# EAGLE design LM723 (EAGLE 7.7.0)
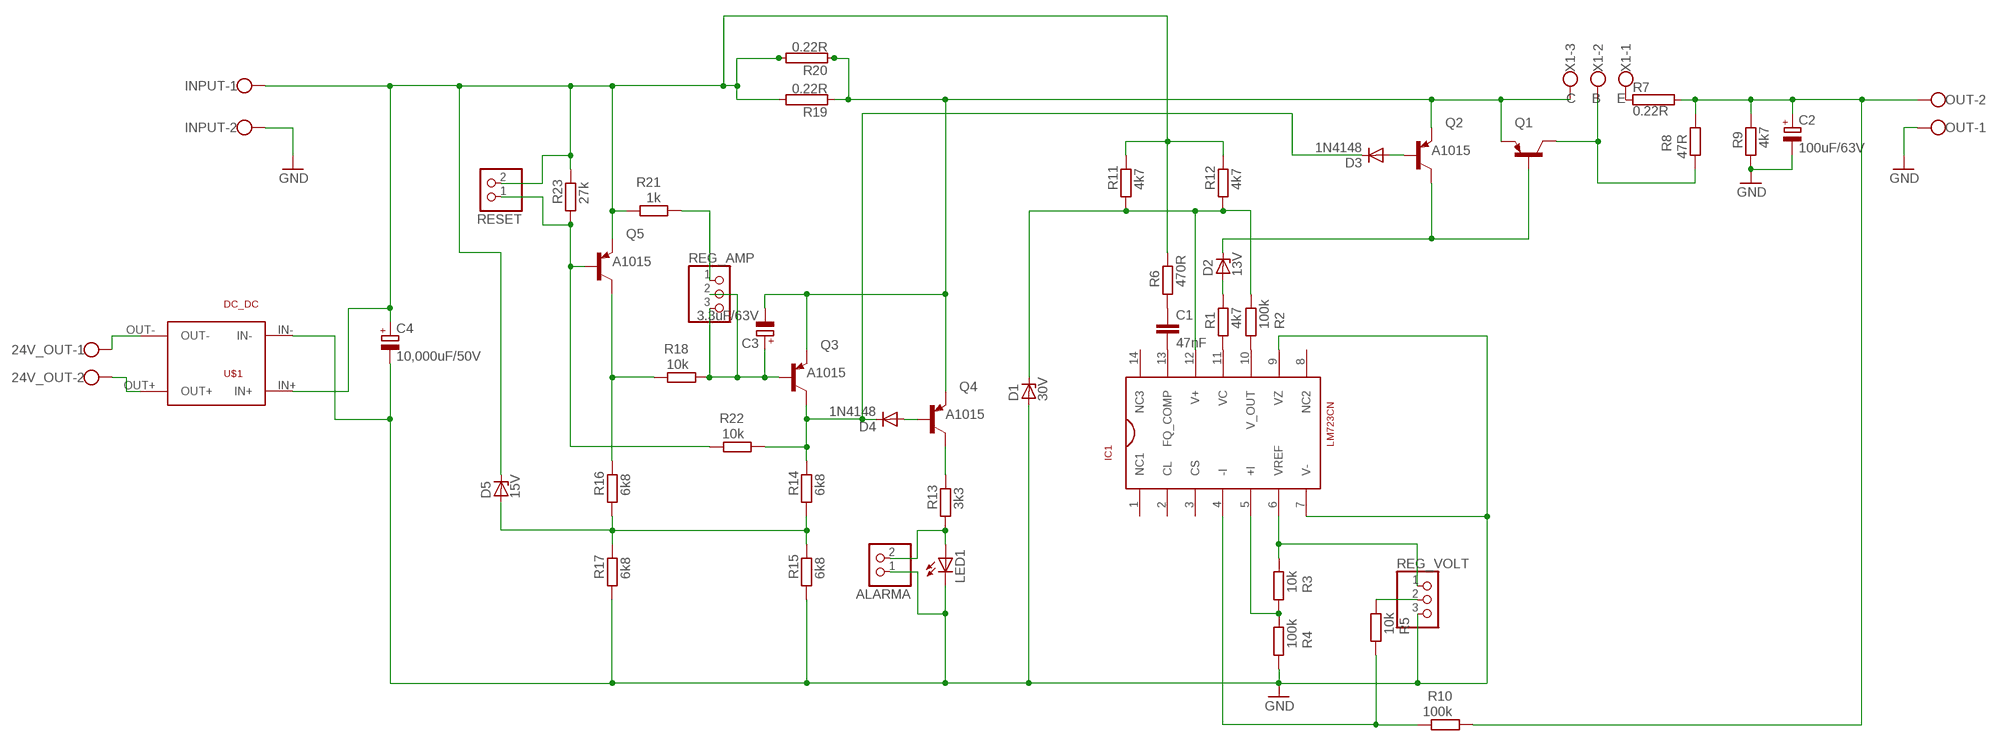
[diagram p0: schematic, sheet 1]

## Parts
24V_OUT  W237-102  [W237-102]
ALARMA  PINHD-1X2  [1X02]
C1  47nF  C-EU050-025X075  [C050-025X075]
C2  100uF/63V  CPOL-EUE5-8.5  [E5-8,5]
C3  3.3uF/63V  CPOL-EUE5-8.5  [E5-8,5]
C4  10,000uF/50V  CPOL-EUE10-35  [EB35D]
D1  30V  BZX55  [DO35Z10]
D2  13V  BZX55  [DO35Z10]
D3  1N4148  1N4148DO35-10  [DO35-10]
D4  1N4148  1N4148DO35-10  [DO35-10]
D5  15V  BZX55  [DO35Z10]
IC1  LM723CN  [DIL14]
INPUT  W237-102  [W237-102]
LED1  LED5MM  [LED5MM]
OUT  W237-102  [W237-102]
Q1  -PNP-TO220V  [TO220V]
Q2  A1015  2N3906  [TO92]
Q3  A1015  2N3906  [TO92]
Q4  A1015  2N3906  [TO92]
Q5  A1015  2N3906  [TO92]
R1  4k7  R-EU_0204/7  [0204/7]
R2  100k  R-EU_0204/7  [0204/7]
R3  10k  R-EU_0204/7  [0204/7]
R4  100k  R-EU_0204/7  [0204/7]
R5  10k  R-EU_0204/7  [0204/7]
R6  470R  R-EU_0204/7  [0204/7]
R7  0.22R  RHPS923  [HPS923]
R8  47R  R-EU_0204/7  [0204/7]
R9  4k7  R-EU_0204/7  [0204/7]
R10  100k  R-EU_0204/7  [0204/7]
R11  4k7  R-EU_0204/7  [0204/7]
R12  4k7  R-EU_0204/7  [0204/7]
R13  3k3  R-EU_0204/7  [0204/7]
R14  6k8  R-EU_0204/7  [0204/7]
R15  6k8  R-EU_0204/7  [0204/7]
R16  6k8  R-EU_0204/7  [0204/7]
R17  6k8  R-EU_0204/7  [0204/7]
R18  10k  R-EU_0204/7  [0204/7]
R19  0.22R  RMNS-5  [MNS-5]
R20  0.22R  RMNS-5  [MNS-5]
R21  1k  R-EU_0204/7  [0204/7]
R22  10k  R-EU_0204/7  [0204/7]
R23  27k  R-EU_0204/7  [0204/7]
REG_AMP  PINHD-1X3  [1X03]
REG_VOLT  PINHD-1X3  [1X03]
RESET  PINHD-1X2  [1X02]
U$1  DC_DC  [DC_DC]
X1  C B E  W237-103  [W237-103]

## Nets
GND: ALARMA.1 C2.- C4.- D1.A IC1.7(V-) IC1.9(VZ) INPUT.2 LED1.K(C) OUT.1 R4.1 R9.1 R15.1 R17.1 REG_VOLT.3 U$1.IN-
INPUT+: C4.+ D5.C INPUT.1 Q5.3(E) R6.2 R11.2 R12.2 R19.2 R20.2 R21.2 R23.2 RESET.2 U$1.IN+
INPUT+R: C3.- Q1.3(E) Q2.3(E) Q3.3(E) Q4.3(E) R19.1 R20.1 X1.3
N$1: IC1.11(VC) R1.1
N$2: IC1.10(V_OUT) R2.1
N$3: IC1.6(VREF) R3.2 REG_VOLT.1
N$4: IC1.5(+I) R3.1 R4.2
N$5: Q1.2(C) R8.2 X1.2
N$6: C1.2 IC1.13(FQ_COMP)
N$7: R5.2 REG_VOLT.2
N$8: C1.1 R6.1
N$10: R21.1 REG_AMP.1
N$11: R7.1 X1.1
N$12: IC1.4(-I) R5.1 R10.2
N$13: D2.C Q1.1(B) Q2.1(C)
N$14: D2.A R1.2
N$15: 24V_OUT.1 U$1.OUT-
N$16: D1.C IC1.12(V+) R2.2 R11.1 R12.1
N$17: Q5.1(C) R16.2 R18.2
N$18: D3.A Q2.2(B)
N$19: D4.A Q4.2(B)
N$20: Q4.1(C) R13.2
N$21: ALARMA.2 LED1.A R13.1
N$22: D3.C D4.C Q3.1(C) R14.2 R22.1
N$23: D5.A R14.1 R15.2 R16.1 R17.2
N$24: C3.+ Q3.2(B) R18.1 REG_AMP.2 REG_AMP.3
N$26: Q5.2(B) R22.2 R23.1 RESET.1
N$27: 24V_OUT.2 U$1.OUT+
OUT+: C2.+ OUT.2 R7.2 R8.1 R9.2 R10.1
Unconnected: IC1.1(NC1) IC1.2(CL) IC1.3(CS) IC1.8(NC2) IC1.14(NC3)

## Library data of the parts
24V_OUT INPUT OUT = con-wago-500:W237-102: WAGO SCREW CLAMP; MPN: 237-102; OC_FARNELL: unknown; OC_NEWARK: 70K9898
ALARMA RESET = pinhead:PINHD-1X2: PIN HEADER
C1 = rcl:C-EU: CAPACITOR, European symbol
C2-C4 = rcl:CPOL-EU: POLARIZED CAPACITOR, European symbol
D1 D2 D5 = diode:BZX55: Z DIODE
D3 D4 = diode:1N4148: DIODE
IC1 = linear:LM723CN
LED1 = led:LED: LED
Q1 = transistor:*-PNP-: PNP Transistror
Q2-Q5 = transistor-pnp:2N3906: PNP Transistor
R1-R6 R8-R18 R21-R23 = rcl:R-EU_: RESISTOR, European symbol
R7 R19 R20 = resistor-power:R: Power Resitor; OC_FARNELL: unknown; OC_NEWARK: unknown
REG_AMP REG_VOLT = pinhead:PINHD-1X3: PIN HEADER
U$1 = Vitico Torres:DC_DC
X1 = con-wago-500:W237-103: WAGO SCREW CLAMP; MPN: 237-103; OC_FARNELL: unknown; OC_NEWARK: 18M7116

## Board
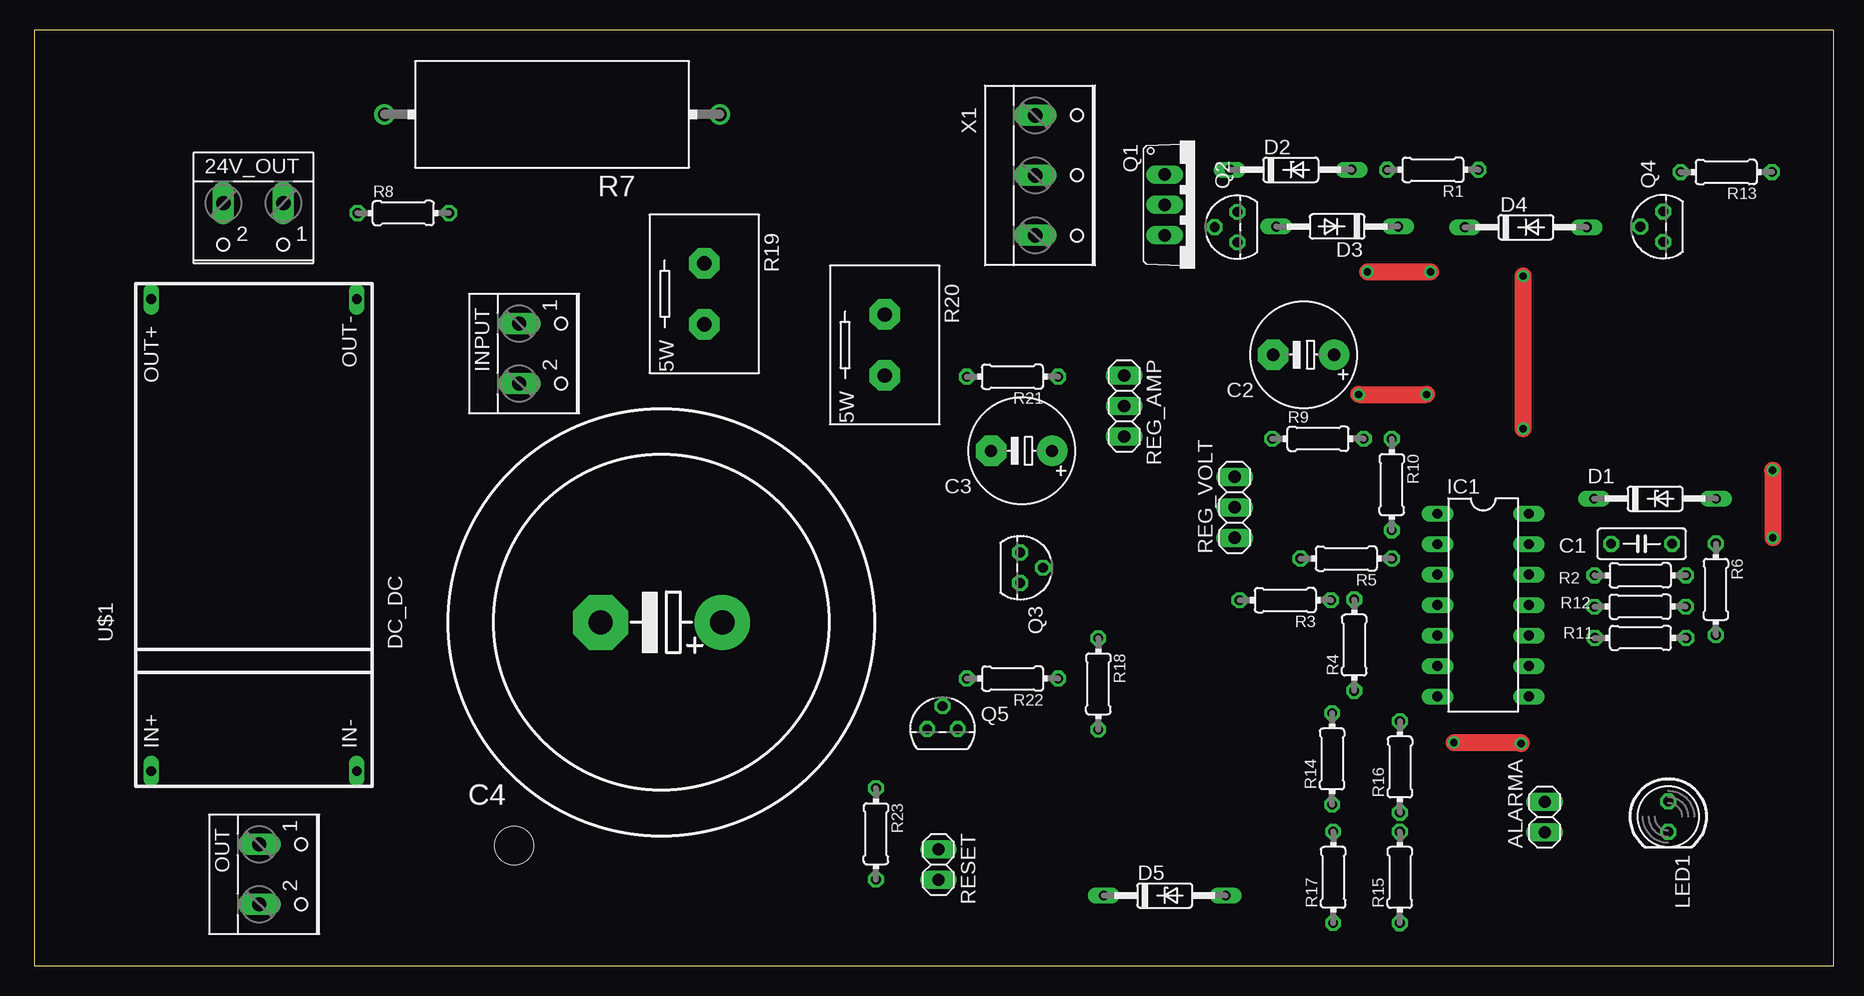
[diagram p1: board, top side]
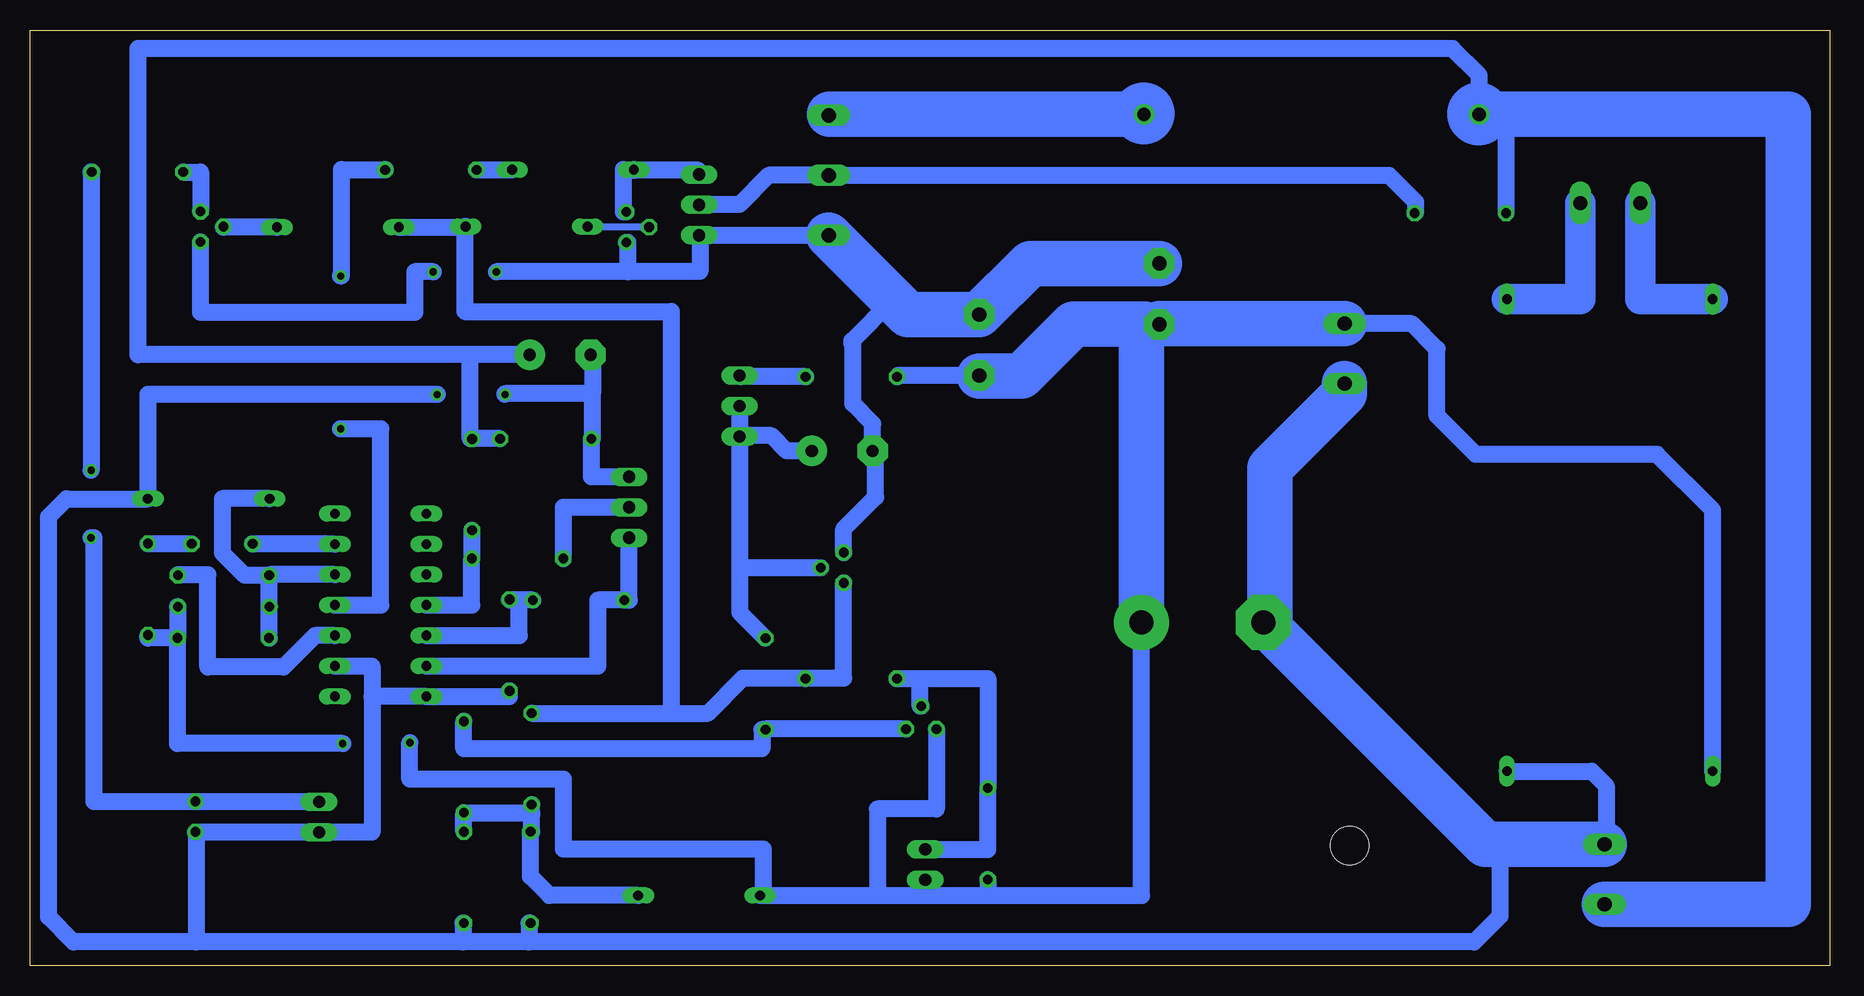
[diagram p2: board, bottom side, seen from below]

Size 150 x 78 mm. Coordinates in mm from the lower left corner, seen from the top.
Outline: 0,0 150,0 150,78 0,78 0,0
Copper layers (1*16): Top 0.035mm / dielectric 1.5mm / Bottom 0.035mm
Design rules "default": minimum track width 10mil, minimum drill 24mil, track to track 8mil, track to pad 8mil, pad to pad 8mil, via to via 8mil, smd to smd 8mil, copper to edge 40mil, drill to drill 8mil, minimum pad ring 10mil, minimum via ring 8mil, stop-mask expansion 4mil, vias tented up to drill 0mil, thermal gap 10mil
Holes 3.2 mm at 40,10

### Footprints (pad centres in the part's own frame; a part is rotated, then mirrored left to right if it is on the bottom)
W237-102 = drill 1.194 long: 1 -2.5,-1.27; 2 2.5,-1.27
1X02 = drill 1.016 long: 1 -1.27,0; 2 1.27,0
C050-025X075 = drill 0.813 octagon: 1 -2.54,0; 2 2.54,0
E5-8,5 = drill 1.016 pad 2.54: + -2.54,0 | drill 1.016 pad 2.54 octagon: - 2.54,0
EB35D = drill 2.007 pad 4.597: + -5.08,0 | drill 2.007 pad 4.597 octagon: - 5.08,0
DO35Z10 = drill 0.813 long: A 5.08,0; C -5.08,0
DO35-10 = drill 0.813 long: A 5.08,0; C -5.08,0
DIL14 = drill 0.813 long: 1 -7.62,-3.81; 2 -5.08,-3.81; 3 -2.54,-3.81; 4 0,-3.81; 5 2.54,-3.81; 6 5.08,-3.81; 7 7.62,-3.81; 8 7.62,3.81; 9 5.08,3.81; 10 2.54,3.81; 11 0,3.81; 12 -2.54,3.81; 13 -5.08,3.81; 14 -7.62,3.81
LED5MM = drill 0.813 octagon: A -1.27,0; K 1.27,0
TO220V = drill 1.016 long: 1 -2.54,-2.54; 2 0,-2.54; 3 2.54,-2.54
TO92 = drill 0.813 octagon: 1 1.27,0; 2 0,1.905; 3 -1.27,0
0204/7 = drill 0.813 octagon: 1 -3.81,0; 2 3.81,0
HPS923 = drill 1.1 pad 1.7: 1 -13.97,0; 2 13.97,0
MNS-5 = drill 1.194 pad 2.54 octagon: 1 -2.54,0; 2 2.54,0
1X03 = drill 1.016 long: 1 -2.54,0; 2 0,0; 3 2.54,0
DC_DC = drill 0.8 long: IN+ -23.495,8.255; IN- -23.495,-8.89; OUT+ 15.875,8.255; OUT- 15.875,-8.89
W237-103 = drill 1.194 long: 1 -5,-1.29; 2 0,-1.29; 3 5,-1.29

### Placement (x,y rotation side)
24V_OUT  18.26,62.3 180 top
ALARMA  125.9,12.39 90 top
C1  133.99,35.16 180 top
C2  105.81,50.92 180 top
C3  82.3,42.9 180 top
C4  52.27,28.61 180 top
D1  135.1,38.93 0 top
D2  104.74,66.35 0 top
D3  108.61,61.61 180 top
D4  124.33,61.55 0 top
D5  94.22,5.84 0 top
IC1  120.78,30.05 270 top
INPUT  41.69,51.02 270 top
LED1  136.21,12.41 270 top
OUT  20.02,7.6 270 top
Q1  96.77,63.42 270 top
Q2  100.3,61.56 90 top
Q3  82.18,33.17 270 top
Q4  135.78,61.6 90 top
Q5  75.71,19.71 0 top
R1  116.58,66.34 180 top
R2  133.86,32.53 180 top
R3  104.27,30.46 180 top
R4  110.03,26.71 90 top
R5  109.36,33.93 180 top
R6  140.17,31.37 270 top
R7  43.17,70.96 180 top
R8  30.76,62.74 0 top
R9  107.01,43.92 0 top
R10  113.15,40.09 270 top
R11  133.89,27.31 0 top
R12  133.86,29.92 0 top
R13  141.04,66.16 180 top
R14  108.18,17.23 90 top
R15  113.83,7.34 90 top
R16  113.84,16.55 90 top
R17  108.27,7.35 90 top
R18  88.69,23.48 270 top
R19  55.86,56 270 top
R20  70.89,51.73 270 top
R21  81.54,49.09 180 top
R22  81.55,23.93 180 top
R23  70.16,10.98 270 top
REG_AMP  90.85,46.64 270 top
REG_VOLT  100.06,38.21 90 top
RESET  75.37,8.41 270 top
U$1  18,39.69 90 top
X1  84.72,65.88 270 top

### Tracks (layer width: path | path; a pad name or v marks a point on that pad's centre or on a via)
GND  (via drill 0.6)
  Top 1.422: v110.4,47.62 v116.05,47.62
  Bottom 1.422: C4.- 46.38,28.61 27.48,9.71 27.48,4.11 29.61,1.98 108.4,1.98 | 108.4,1.98 113.9,1.98 | 113.9,1.98 136.15,1.98 | 136.15,1.98 146.38,1.98 148.45,4.04 148.45,37.42 146.97,38.91 140.2,38.91 D1.A | U$1.IN- 19.83,16.2 18.61,14.97 18.61,10.25 OUT.1 | 140.18,39.02 D1.A | R17.1 108.4,3.54 108.4,1.98 | R15.1 113.9,3.53 113.9,1.98 | 136.15,1.98 136.15,11.14 LED1.K 136.21,11.12 ALARMA.1 121.48,11.12 121.48,22.43 | IC1.9 121.48,24.98 121.48,22.43 | 121.48,22.43 IC1.7 110.03,22.43 R4.1 | C2.- 103.12,50.92 103.12,47.69 | 103.12,47.69 110.4,47.69 v110.4,47.62 | v116.05,47.62 140.18,47.62 D1.A | REG_VOLT.3 103.2,40.75 R9.1 103.12,43.92 103.12,47.69
  Bottom 3.81: OUT.1 28.68,10.1 C4.- 46.65,29.16 46.65,41.46 40.42,47.69 INPUT.2
INPUT+  (via drill 0.6)
  Top 1.422: v118.34,18.59 123.94,18.59 v123.94,18.51
  Bottom 1.422: R12.2 137.7,29.92 R11.2 | R11.2 140.17,27.31 R6.2 | 79.36,5.84 D5.C 88.86,5.84 88.86,9.69 105.53,9.69 105.53,15.54 118.34,15.54 v118.34,18.59 | 79.36,5.84 75.28,5.84 | 75.28,5.84 70.16,5.84 | 70.16,5.84 57.35,5.84 C4.+ | Q5.3 74.46,19.71 74.46,13.05 79.36,13.05 79.36,5.84 | RESET.2 75.28,7.14 75.28,5.84 | R23.2 70.16,5.84 | v123.94,18.51 137.7,18.51 R11.2 | R20.2 77.63,49.19 R21.2 | U$1.IN+ 9.74,37.98 14.38,42.61 29.48,42.61 32.72,45.84 32.72,51.4 34.83,53.51 INPUT.1
  Bottom 2.6: R19.2 57.07,53.46 57.35,53.18 | 70.84,49.15 R20.2
  Bottom 3.81: 57.07,53.46 63.03,53.46 67.34,49.15 70.84,49.15 | C4.+ 57.35,53.18 | INPUT.1 55.86,53.52 R19.2
INPUT+R  (via drill 0.6)
  Top 1.422: v111.13,57.84 v116.39,57.84
  Bottom 1.422: X1.3 Q1.3 94.17,60.88 94.17,57.87 100.19,57.87 | Q3.3 82.18,36.39 79.51,39.05 79.51,42.65 C3.- 79.76,45.18 81.42,46.84 81.42,51.79 81.49,51.86 81.49,52.08 78.06,55.51 | Q2.3 100.19,60.29 100.19,57.87 | v111.13,57.84 100.19,57.84 100.19,57.87 | v116.39,57.84 117.92,57.84 117.92,54.44 135.78,54.44 Q4.3
  Bottom 3.81: R19.1 66.62,58.54 R20.1 76.82,54.27 78.06,55.51 X1.3
N$1  (via drill 0.6)
  Top 1.422: v124.11,44.75 v124.11,57.49
  Bottom 1.422: IC1.11 120.75,30.05 120.75,44.75 v124.11,44.75 | v124.11,57.49 124.02,57.49 124.02,66.36 120.39,66.36 R1.1
N$2
  Bottom 1.422: IC1.10 126.24,27.52 128.87,24.89 135.18,24.89 135.18,32.58 137.67,32.58 R2.1
N$3
  Bottom 1.422: IC1.6 102.65,24.98 102.65,30.46 R3.2 100.06,30.46 REG_VOLT.1
N$4
  Bottom 1.422: R3.1 109.21,30.46 | 109.21,30.46 109.97,30.46 R4.2 | IC1.5 109.21,27.52 109.21,30.46
N$5
  Bottom 1.422: Q1.2 94.21,63.44 90.87,63.44 88.43,65.88 X1.2 36.72,65.88 34.51,63.67 34.51,62.8 R8.2
N$6
  Bottom 1.422: IC1.13 131.42,35.13 C1.2
N$7
  Bottom 1.422: REG_VOLT.2 105.55,38.21 R5.2
N$8
  Bottom 1.422: C1.1 140.15,35.16 R6.1
N$10
  Bottom 1.422: R21.1 90.77,49.09 REG_AMP.1
N$11
  Bottom 2.6: 83.35,70.96 X1.1
  Bottom 3.81: R7.1 83.35,70.96
N$12
  Bottom 1.422: IC1.4 113.17,30.05 R5.1 113.15,33.93 R10.2
N$13
  Bottom 1.422: Q1.1 94.28,65.96 94.28,66.3 99.66,66.3 D2.C 100.53,66.36 100.53,62.83 Q2.1
N$14
  Bottom 1.422: R1.2 D2.A
N$15
  Bottom 2.54: U$1.OUT- 20.77,55.57 24V_OUT.1
N$16
  Bottom 1.422: IC1.12 129.99,32.59 R2.2 | R11.1 130.04,27.31 R12.1 R2.2 | R2.2 132.09,32.53 133.96,34.4 133.96,38.93 D1.C
N$17
  Bottom 1.422: Q5.1 88.69,19.71 R18.2 88.99,19.67 88.99,18.08 113.84,18.08 R16.2
N$18
  Bottom 0.254: 103.53,61.56 D3.A
  Bottom 0.6: Q2.2 103.53,61.56
N$19
  Bottom 1.422: D4.A 133.88,61.55 Q4.2
N$20
  Bottom 1.422: R13.2 135.78,66.16 Q4.1
N$21  (via drill 0.6)
  Top 1.422: v144.9,41.29 144.92,41.29 v144.92,35.67
  Bottom 1.422: R13.1 144.9,66.16 v144.9,41.29 | v144.92,35.67 144.68,35.67 144.68,13.68 LED1.A 136.21,13.66 ALARMA.2
N$22
  Bottom 1.422: R14.2 96.55,21.04 | 96.55,21.04 93.5,21.04 90.57,23.97 85.4,23.97 | 85.4,23.97 R22.1 | 96.55,21.04 96.55,54.52 113.76,54.52 113.76,61.61 D3.C 113.69,61.55 D4.C | 85.4,23.97 82.18,23.97 Q3.1
N$23
  Bottom 1.422: D5.A 106.69,5.84 108.28,7.43 R17.2 108.19,11.16 108.19,12.6 108.19,12.74 | 108.19,12.74 R14.1 | R15.2 R16.1 108.19,12.74
N$24
  Bottom 1.422: REG_AMP.3 90.85,32.97 | 90.85,32.97 90.85,29.45 R18.1 | Q3.2 90.66,33.17 90.85,32.97 | C3.+ 86.94,42.9 88.21,44.17 90.78,44.17 REG_AMP.3 | REG_AMP.2 REG_AMP.3
N$26
  Bottom 1.422: RESET.1 70.16,9.69 R23.1 70.16,23.93 75.81,23.93 | R22.2 75.81,23.93 | Q5.2 75.81,21.62 75.81,23.93
N$27
  Bottom 2.54: U$1.OUT+ 15.77,55.57 24V_OUT.2
OUT+
  Bottom 1.422: 29.2,70.98 R7.2 29.2,74.22 31.42,76.44 141,76.44 141,50.92 113.3,50.92 | R8.1 26.95,70.52 27.39,70.96 | C2.+ 113.3,50.92 | R9.2 113.15,43.92 R10.1 113.3,43.9 113.3,50.92
  Bottom 2.54: OUT.2
  Bottom 3.81: R7.2 27.39,70.96 3.45,70.96 3.45,5.11 OUT.2
(copper drawn outside any net)
  shapes: Bottom circle x2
